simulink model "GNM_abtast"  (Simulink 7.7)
settings: Solver=ode45  StartTime=0.0  StopTime=0.2  RelTol=1e-3
InitFcn:
  | GNM_abtast_ini
StopFcn:
  | GNM_abtast_plot
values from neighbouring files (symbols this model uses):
  CE = 240.02    [GNM_abtast_ini.m]
  CM = CE/2/pi    (= 38.2003694409)    [GNM_abtast_ini.m]
  Fpwm = 5000    [GNM_abtast_ini.m]
  IAmax = 20    [GNM_abtast_ini.m]
  J = 0.012    [GNM_abtast_ini.m]
  LA = 0.004    [GNM_abtast_ini.m]
  Mw = 10    [GNM_abtast_ini.m]
  N_soll = 1000 / 60    (= 16.6666666667)    [GNM_abtast_ini.m]
  psi = 0.04    [GNM_abtast_ini.m]
  RA = 0.25    [GNM_abtast_ini.m]
  TRN = 8*Tstr    (= 0.0032)    [GNM_abtast_ini.m]
  Ts = 0.0008    [GNM_abtast_ini.m]
  Umax = 200    [GNM_abtast_ini.m]
  VRN = 2*pi*J/(4*Tstr*CM*psi)    (= 30.8399437581)    [GNM_abtast_ini.m]
undefined symbols (not defined in the file or in its folder): Ad, Bd
libraries: simulink x1

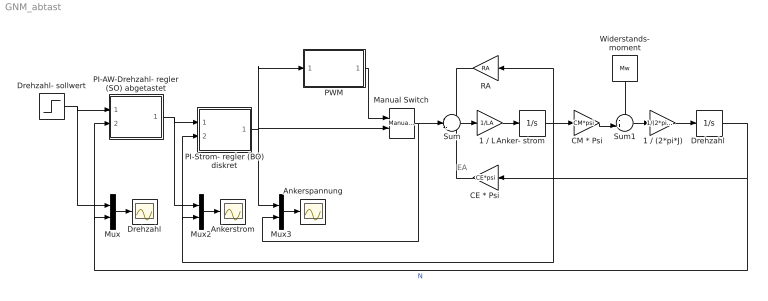
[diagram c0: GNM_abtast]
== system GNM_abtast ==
  note: EA
  " Widerstands-  moment" : Constant  Value=Mw
  1 / (2*pi*J) : Gain  Gain=1/(2*pi*J)
  1 / LA : Gain  Gain=1/LA
  Anker- strom : Integrator
  Ankerspannung : Scope
  Ankerstrom : Scope
  "CE * Psi " : Gain  Gain=CE*psi
  CM * Psi : Gain  Gain=CM*psi
  Drehzahl : Scope
  "Drehzahl " : Integrator
  Drehzahl- sollwert : Step  Time=0.05  After=N_soll  SampleTime=0
  Manual Switch : simulink/Signal Routing/Manual Switch  SystemSampleTime=-1  sw=0  action=0  varsize=off
  Mux : Mux  Inputs=2
  Mux2 : Mux  Inputs=2
  Mux3 : Mux  Inputs=2
  PI-AW-Drehzahl- regler (SO) abgetastet : Subsystem
  PI-Strom- regler (BO) diskret : Subsystem
  PWM : Subsystem
  RA : Gain  Gain=RA
  Sum : Sum  Inputs=-+-
  Sum1 : Sum  Inputs=-+|
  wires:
  RA/1 -> Sum/1
  Anker- strom/1 -> CM * Psi/1, RA/1, Mux2/2, PI-Strom- regler (BO) diskret/2(IA)
  Sum/1 -> 1 / LA/1
  1 / LA/1 -> Anker- strom/1
  CM * Psi/1 -> Sum1/2
  Sum1/1 -> 1 / (2*pi*J)/1
  1 / (2*pi*J)/1 -> "Drehzahl "/1
  " Widerstands-  moment"/1 -> Sum1/1
  "CE * Psi "/1 -> Sum/3
  PWM/1(UAist) -> Manual Switch/1
  Mux/1 -> Drehzahl/1
  PI-AW-Drehzahl- regler (SO) abgetastet/1(IAsoll) -> PI-Strom- regler (BO) diskret/1(IAsoll), Mux2/1
  Mux2/1 -> Ankerstrom/1
  Mux3/1 -> Ankerspannung/1
  PI-Strom- regler (BO) diskret/1(UAsoll) -> Mux3/1, PWM/1(UAsoll), Manual Switch/2
  Drehzahl- sollwert/1 -> Mux/1, PI-AW-Drehzahl- regler (SO) abgetastet/1(N_soll)
  Manual Switch/1 -> Sum/2, Mux3/2
  "Drehzahl "/1 -> "CE * Psi "/1, Mux/2, PI-AW-Drehzahl- regler (SO) abgetastet/2(N)  "N"

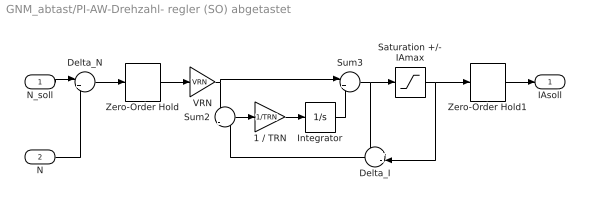
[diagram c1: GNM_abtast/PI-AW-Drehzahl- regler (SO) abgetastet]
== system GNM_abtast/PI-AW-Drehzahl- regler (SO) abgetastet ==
  N_soll : Inport
  N : Inport  Port=2
  1 / TRN : Gain  Gain=1/TRN
  Delta_I : Sum  Inputs=+-|
  Delta_N : Sum  Inputs=|+-
  Integrator : Integrator
  Saturation +/- IAmax : Saturate  UpperLimit=IAmax  LowerLimit=-IAmax
  Sum2 : Sum  Inputs=+|-
  Sum3 : Sum  Inputs=|++
  VRN : Gain  Gain=VRN
  Zero-Order Hold : ZeroOrderHold  SampleTime=Ts
  Zero-Order Hold1 : ZeroOrderHold  SampleTime=Ts
  IAsoll : Outport  InitialOutput=0
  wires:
  N_soll/1 -> Delta_N/1
  N/1 -> Delta_N/2
  Delta_N/1 -> Zero-Order Hold/1
  Integrator/1 -> Sum3/2
  Sum3/1 -> Saturation +/- IAmax/1, Delta_I/1
  Sum2/1 -> 1 / TRN/1
  VRN/1 -> Sum2/1, Sum3/1
  Delta_I/1 -> Sum2/2
  1 / TRN/1 -> Integrator/1
  Saturation +/- IAmax/1 -> Delta_I/2, Zero-Order Hold1/1
  Zero-Order Hold/1 -> VRN/1
  Zero-Order Hold1/1 -> IAsoll/1

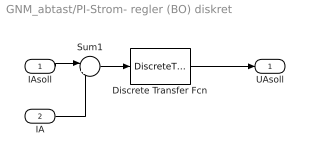
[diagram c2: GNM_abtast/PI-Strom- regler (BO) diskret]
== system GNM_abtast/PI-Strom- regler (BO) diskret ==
  IAsoll : Inport
  IA : Inport  Port=2
  Discrete Transfer Fcn : DiscreteTransferFcn  Numerator=Bd  Denominator=Ad  SampleTime=Ts
  Sum1 : Sum  Inputs=|+-
  UAsoll : Outport  InitialOutput=0
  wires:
  IAsoll/1 -> Sum1/1
  IA/1 -> Sum1/2
  Sum1/1 -> Discrete Transfer Fcn/1
  Discrete Transfer Fcn/1 -> UAsoll/1

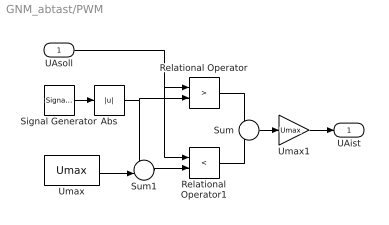
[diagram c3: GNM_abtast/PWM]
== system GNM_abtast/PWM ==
  UAsoll : Inport
  Abs : Abs
  Relational Operator : RelationalOperator  Operator=>
  Relational Operator1 : RelationalOperator  Operator=<
  Signal Generator : SignalGenerator  WaveForm=sawtooth  Amplitude=Umax  Frequency=Fpwm
  Sum : Sum  Inputs=+-
  Sum1 : Sum  Inputs=+-|
  Umax : Constant  Value=Umax
  Umax1 : Gain  Gain=Umax
  UAist : Outport  InitialOutput=0
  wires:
  Signal Generator/1 -> Abs/1
  Sum1/1 -> Relational Operator1/2
  UAsoll/1 -> Relational Operator1/1, Relational Operator/1
  Abs/1 -> Relational Operator/2, Sum1/1
  Umax/1 -> Sum1/2
  Relational Operator/1 -> Sum/1
  Relational Operator1/1 -> Sum/2
  Umax1/1 -> UAist/1
  Sum/1 -> Umax1/1
